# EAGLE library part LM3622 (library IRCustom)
National LM3622 li-ion charger http://www.ladyada.net/library/eagle
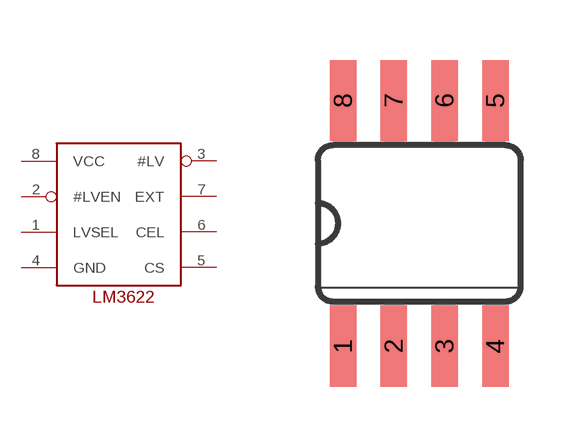
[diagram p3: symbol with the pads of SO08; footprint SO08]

Designator prefix -

## LM3622  [SO08]
1  LVSEL  in
2  #LVEN  in
3  #LV  out
4  GND  sup
5  CS  pas
6  CEL  pas
7  EXT  out
8  VCC  sup

## Footprint SO08 (pad centres in mm)
smd 0.66 x 2.032: 1 -1.905,-3.073; 2 -0.635,-3.073; 3 0.635,-3.073; 4 1.905,-3.073; 5 1.905,3.073; 6 0.635,3.073; 7 -0.635,3.073; 8 -1.905,3.073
